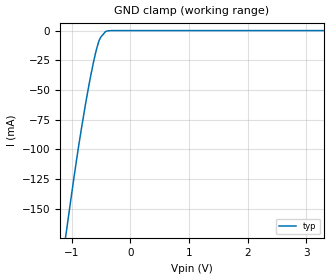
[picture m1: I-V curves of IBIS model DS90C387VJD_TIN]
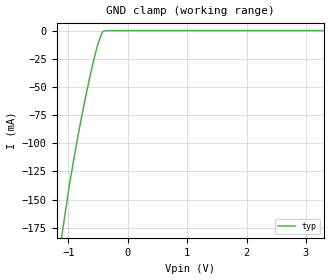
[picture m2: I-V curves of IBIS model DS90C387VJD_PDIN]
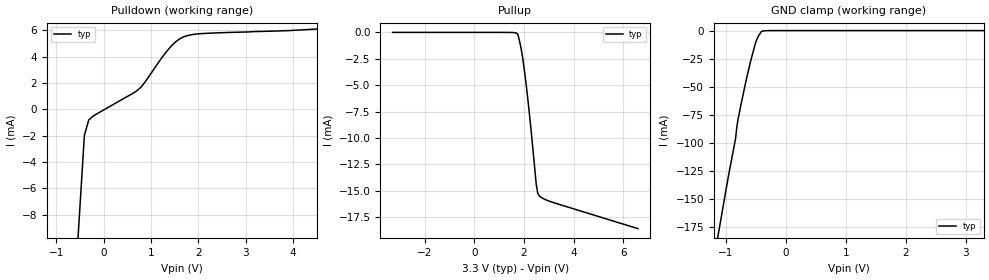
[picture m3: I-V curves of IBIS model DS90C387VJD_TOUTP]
|   National Semiconductor Corporation
|   Interface Products Group
|   IBIS Model of Channel Link Transmitter
|   100VJD TQFP
[IBIS Ver]   2.1
[Comment char]  |_char
[File name]   c387vjd.ibs
[File Rev]   2.0
[Date]   1/10/2000
[Source]   File originated at National Semiconductor Corporation.
   Interface Group/Analog Division. All data based on
   Empirical Measurements(Bench).
[Notes]   File created by CW.
   Revision 1: The original model
   Revision 2: Change "vdiff" values from "NA" to 0.1;
   Corrected "Ramp" rate data.
[Disclaimer]
(C) Copyright National Semiconductor Corporation 1999
   All rights reserved
   National Semiconductor Corporation hereby grants
the user of this IBIS model a non-exclusive, nontransferable
license to use this IBIS model under the following terms.
Before using this IBIS model, the user should read this
license.  If the user does not accept these terms,  the
IBIS model should be returned to National within 30 days.
   The user is granted this license only to use the
IBIS model and is not granted rights to sell, load, rent,
lease or license the IBIS model in whole or in part, or in
modified form to anyone other than user. User may modify
the IBIS model to suit its specific applications but rights
to derivative works and such modifications shall belong to
National.
   This IBIS model is provided on an "AS IS" basis and
National makes absolutely no warranty with respect to the
information contained herein. NATIONAL DISCLAIMS AND CUSTOMER
WAIVES ALL WARRANTIES, EXPRESS OR IMPLIED, INCLUDING
WARRANTIES OF MERCHANTABILITY OR FITNESS FOR A PARTICULAR
PURPOSE. The entire risk as to quality and performance is
with the Customer. ACCORDINGLY, IN NO EVENT SHALL THE
COMPANY BE LIABLE FOR ANY DAMAGES, WHETHER IN CONTRACT OR
TORT,INCLUDING ANY LOST PROFITS OR OTHER INCIDENTAL,
CONSEQUENTIAL, EXEMPLARY, OR PUNITIVE DAMAGES ARISING OUT
OF THE USE OR APPLICATION OF THE IBIS model provided in
this package. Further, National reserves the right to make
changes without notice to any product herein to improve
reliability, function, or design. National does not convey
any license under patent rights or any other intellectual
property rights, including those of third parties.
   National is not obligated to provide maintenance or support
for the licensed IBIS model.
Contact National at ATTN:INTERFACE APPLICATIONS/IBIS MODELS.
2900 Semiconductor Drive, M/S A2595, Santa Clara, CA 95052-8090
|!!!Please note pre-emphasis feature is NOT modeled!!!
[Copyright]   Copyright 1999, National Semiconductor, All Rights Reserved
[Component]   DS90C387VJD
[Manufacturer]  National Semiconductor Corp
[Package]
|   typ   min   max
R_pkg   64.20m   NA   NA
L_pkg   2.491nH   NA   NA
C_pkg   0.3380pF   NA   NA
[Pin]   signal_name   model_name   R_pin   L_pin   C_pin
1   TxING11   DS90C387VJD_TIN   70.72m  2.917n   0.3789p
2   TxING10   DS90C387VJD_TIN   70.51m  2.771n   0.3776p
3   TxINR17   DS90C387VJD_TIN   68.62m  2.713n   0.3658p
4   TxINR16   DS90C387VJD_TIN   67.20m  2.650n   0.3568p
5   TxINR15   DS90C387VJD_TIN   65.58m  2.545n   0.3467p
6   TxINR14   DS90C387VJD_TIN   64.85m  2.496n   0.3421p
7   TxINR13   DS90C387VJD_TIN   63.40m  2.419n   0.3328p
8   TxINR12   DS90C387VJD_TIN   62.50m  2.437n   0.3272p
9   TxINR11   DS90C387VJD_TIN   61.19m  2.376n   0.3192p
10   TxINR10   DS90C387VJD_TIN   60.16m  2.276n   0.3127p
11   TxCLKIN   DS90C387VJD_TIN   59.45m  2.239n   0.3083p
12   PLLVCC   POWER   58.73m  2.205n   0.3038p
13   GND   GND   59.19m  2.179n   0.3067p
14   PRE   DS90C387VJD_PDIN   58.73m  2.205n   0.3038p
15   PLLSEL   DS90C387VJD_PDIN   59.45m  2.239n   0.3083p
16   PLLGND   GND   60.16m  2.276n   0.3127p
17   PLLGND   GND   61.19m  2.376n   0.3192p
18   PLLVCC   POWER   62.50m  2.437n   0.3272p
19   PLLGND   GND   63.40m  2.419n   0.3328p
20   R_FB   DS90C387VJD_PDIN   64.85m  2.496n   0.3421p
21   R_FDE   DS90C387VJD_PDIN   65.58m  2.545n   0.3467p
22   PD*   DS90C387VJD_PDIN   67.20m  2.650n   0.3568p
23   DUAL   DS90C387VJD_PDIN   68.62m  2.713n   0.3658p
24   BAL   DS90C387VJD_PDIN   70.51m  2.771n   0.3776p
25   LVDSGND   GND   70.72m  2.917n   0.3789p
26   TxCLKOUT2+   DS90C387VJD_TOUTP   70.72m  2.917n   0.3789p
27   TxCLKOUT2-   DS90C387VJD_TOUTM   70.51m  2.771n   0.3776p
28   TxOUTA7+   DS90C387VJD_TOUTP   68.62m  2.713n   0.3658p
29   TxOUTA7-   DS90C387VJD_TOUTM   67.20m  2.650n   0.3568p
30   LVDSVCC   POWER   65.58m  2.545n   0.3467p
31   TxOUTA6+   DS90C387VJD_TOUTP   64.85m  2.496n   0.3421p
32   TxOUTA6-   DS90C387VJD_TOUTM   63.40m  2.419n   0.3328p
33   TxOUTA5+   DS90C387VJD_TOUTP   62.50m  2.437n   0.3272p
34   TxOUTA5-   DS90C387VJD_TOUTM   61.19m  2.376n   0.3192p
35   LVDSGND   GND   60.16m  2.276n   0.3127p
36   TxOUTA4+   DS90C387VJD_TOUTP   59.45m  2.239n   0.3083p
37   TxOUTA4-   DS90C387VJD_TOUTM   58.73m  2.205n   0.3038p
38   TxOUTA3+   DS90C387VJD_TOUTP   59.19m  2.179n   0.3067p
39   TxOUTA3-   DS90C387VJD_TOUTM   58.73m  2.205n   0.3038p
40   LVDSVCC   POWER   59.45m  2.239n   0.3083p
41   TxCLKOUT1+   DS90C387VJD_TOUTP   60.16m  2.276n   0.3127p
42   TxCLKOUT1-   DS90C387VJD_TOUTM   61.19m  2.376n   0.3192p
43   LVDSGND   GND   62.50m  2.437n   0.3272p
44   TxOUTA2+   DS90C387VJD_TOUTP   63.40m  2.419n   0.3328p
45   TxOUTA2-   DS90C387VJD_TOUTM   64.85m  2.496n   0.3421p
46   TxOUTA1+   DS90C387VJD_TOUTP   65.58m  2.545n   0.3467p
47   TxOUTA1-   DS90C387VJD_TOUTM   67.20m  2.650n   0.3568p
48   LVDSVCC   POWER   68.62m  2.713n   0.3658p
49   TxOUTA0+   DS90C387VJD_TOUTP   70.51m  2.771n   0.3776p
50   TxOUTA0-   DS90C387VJD_TOUTM   70.72m  2.917n   0.3789p
51   LVDSGND   GND   70.72m  2.917n   0.3789p
52   GND   GND   70.51m  2.771n   0.3776p
53   VCC   POWER   68.62m  2.713n   0.3658p
54   HSYNC   DS90C387VJD_TIN   67.20m  2.650n   0.3568p
55   VSYNC   DS90C387VJD_TIN   65.58m  2.545n   0.3467p
56   DE   DS90C387VJD_TIN   64.85m  2.496n   0.3421p
57   TxINB27   DS90C387VJD_TIN   63.40m  2.419n   0.3328p
58   TxINB26   DS90C387VJD_TIN   62.50m  2.437n   0.3272p
59   TxINB25   DS90C387VJD_TIN   61.19m  2.376n   0.3192p
60   TxINB24   DS90C387VJD_TIN   60.16m  2.276n   0.3127p
61   TxINB23   DS90C387VJD_TIN   59.45m  2.239n   0.3083p
62   TxINB22   DS90C387VJD_TIN   58.73m  2.205n   0.3038p
63   TxINB21   DS90C387VJD_TIN   59.19m  2.179n   0.3067p
64   TxINB20   DS90C387VJD_TIN   58.73m  2.205n   0.3038p
65   TxING27   DS90C387VJD_TIN   59.45m  2.239n   0.3083p
66   TxING26   DS90C387VJD_TIN   60.16m  2.276n   0.3127p
67   VCC   POWER   61.19m  2.376n   0.3192p
68   GND   GND   62.50m  2.437n   0.3272p
69   TxING25   DS90C387VJD_TIN   63.40m  2.419n   0.3328p
70   TxING24   DS90C387VJD_TIN   64.85m  2.496n   0.3421p
71   TxING23   DS90C387VJD_TIN   65.58m  2.545n   0.3467p
72   TxING22   DS90C387VJD_TIN   67.20m  2.650n   0.3568p
73   TxING21   DS90C387VJD_TIN   68.62m  2.713n   0.3658p
74   TxING20   DS90C387VJD_TIN   70.51m  2.771n   0.3776p
75   TxINR27   DS90C387VJD_TIN   70.72m  2.917n   0.3789p
76   TxINR26   DS90C387VJD_TIN   70.72m  2.917n   0.3789p
77   TxINR25   DS90C387VJD_TIN   70.51m  2.771n   0.3776p
78   TxINR24   DS90C387VJD_TIN   68.62m  2.713n   0.3658p
79   TxINR23   DS90C387VJD_TIN   67.20m  2.650n   0.3568p
80   TxINR22   DS90C387VJD_TIN   65.58m  2.545n   0.3467p
81   TxINR21   DS90C387VJD_TIN   64.85m  2.496n   0.3421p
82   VCC   POWER   63.40m  2.419n   0.3328p
83   GND   GND   62.50m  2.437n   0.3272p
84   TxINR20   DS90C387VJD_TIN   61.19m  2.376n   0.3192p
85   TxINB17   DS90C387VJD_TIN   60.16m  2.276n   0.3127p
86   TxINB16   DS90C387VJD_TIN   59.45m  2.239n   0.3083p
87   TxINB15   DS90C387VJD_TIN   58.73m  2.205n   0.3038p
88   TxINB14   DS90C387VJD_TIN   59.19m  2.179n   0.3067p
89   TxINB13   DS90C387VJD_TIN   58.73m  2.205n   0.3038p
90   TxINB12   DS90C387VJD_TIN   59.45m  2.239n   0.3083p
91   TxINB11   DS90C387VJD_TIN   60.16m  2.276n   0.3127p
92   TxINB10   DS90C387VJD_TIN   61.19m  2.376n   0.3192p
93   TxING17   DS90C387VJD_TIN   62.50m  2.437n   0.3272p
94   TxING16   DS90C387VJD_TIN   63.40m  2.419n   0.3328p
95   TxING15   DS90C387VJD_TIN   64.85m  2.496n   0.3421p
96   TxING14   DS90C387VJD_TIN   65.58m  2.545n   0.3467p
97   VCC   POWER   67.20m  2.650n   0.3568p
98   GND   GND   68.62m  2.713n   0.3658p
99   TxING13   DS90C387VJD_TIN   70.51m  2.771n   0.3776p
100   TxING12   DS90C387VJD_TIN   70.72m  2.917n   0.3789p
[Diff_pin]   inv_pin   vdiff   tdelay_typ   tdelay_min   tdelay_max
| The '+' pin is Diff_pin and the '-' pin is the inv_pin
26   27   0.1   0 0 0
28   29   0.1   0 0 0
31   32   0.1   0 0 0
33   34   0.1   0 0 0
36   37   0.1   0 0 0
38   39   0.1   0 0 0
41   42   0.1   0 0 0
44   45   0.1   0 0 0
46   47   0.1   0 0 0
49   50   0.1   0 0 0
| Models and submodels in the file (4): DS90C387VJD_TIN (Input), DS90C387VJD_PDIN (Input), DS90C387VJD_TOUTP (3-state), DS90C387VJD_TOUTM (3-state)
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|   Driver Input  MODEL
[Model]   DS90C387VJD_TIN
Model_type   Input
|Signals   TxINR10 ~ TxINR17, TxINR20 ~ TxINR27, TxING10 ~ TxING17,
|   TxING20 ~ TxING27, TxING10 ~ TxING17, TxING20 ~ TxING27,
|   TxCLKIN, HSYNC, VSYNC, DE, PRE, PLLSEL, R_FB, R_FDE, DUAL, BAL
Vinh = 2.0
Vinl = 0.8
|   typ   min   max
C_comp   5.217pF   NA   NA
|   typ   min   max
[Temperature Range]   25.0   NA   NA
[Voltage range]   3.3V   3.0V   3.6V
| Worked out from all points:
|   GND clamp passes 1 mA (typ) near -0.43 V on its own axis
[Power_clamp]
| Note that the[POWER_clamp]voltage table is referenced to Vcc
| and is calculated using Vtable=Vcc - Vmeasured.
|Voltage   I(typ)   I(min)   I(max)
-3V       0A         NA         NA
3V        0A         NA         NA
[GND_clamp]
|Voltage   I(typ)   I(min)   I(max)
-3.3V     -946.6mA   NA         NA
-1.001V   -136.5mA   NA         NA
-920.1mV  -108.8mA   NA         NA
-838.9mV  -83.09mA   NA         NA
-736.2mV  -53.35mA   NA         NA
-675.7mV  -37.16mA   NA         NA
-634.4mV  -27.34mA   NA         NA
-572.4mV  -14.46mA   NA         NA
-531.6mV  -7.937mA   NA         NA
-429.8mV  -1.026mA   NA         NA
-285.7mV  -7.334uA   NA         NA
3.3V      -100.8nA   NA         NA
|   Driver PWRDWN* Input  MODEL
[Model]   DS90C387VJD_PDIN
Model_type   Input
|Signals   PD*
Vinh = 2.0
Vinl = 0.8
|   typ   min   max
C_comp   5.277pF   NA   NA
|   typ   min   max
[Temperature Range]   25.0   NA   NA
[Voltage range]   3.3V   3.0V   3.6V
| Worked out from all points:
|   GND clamp passes 1 mA (typ) near -0.42 V on its own axis
[Power_clamp]
| Note that the[POWER_clamp]voltage table is referenced to Vcc
| and is calculated using Vtable=Vcc - Vmeasured.
|Voltage   I(typ)   I(min)   I(max)
-3V       0A         NA         NA
3V        0A         NA         NA
[GND_clamp]
|Voltage   I(typ)   I(min)   I(max)
-3.3V     -959.1mA   NA         NA
-1V       -143mA     NA         NA
-982mV    -136.5mA   NA         NA
-920.1mV  -117.4mA   NA         NA
-818.3mV  -87.77mA   NA         NA
-715.5mV  -60.23mA   NA         NA
-613.7mV  -35.12mA   NA         NA
-552.2mV  -21.69mA   NA         NA
-490.3mV  -9.998mA   NA         NA
-428.8mV  -1.679mA   NA         NA
-408.2mV  -422.1uA   NA         NA
3.3V      0A         NA         NA
|   Driver Output(+)  MODEL
[Model]   DS90C387VJD_TOUTP
Model_type   3-state
| Signals   TxOUTA0+ ~ TxOUTA7+; TxCLKOUT1+; TxCLKOUT2+
Vmeas = 1.2V   |This is 0.0v differential on ouput
Cref = 5pF   |Timing specification test load capacitance value
Rref = 50
Vref = 1.2
| variable   typ   min   max
C_comp   5.074pF   NA   NA
|   typ   min   max
[Temperature Range]   25.0   NA   NA
[Voltage range]   3.3V   3.0V   3.6V
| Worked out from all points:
|   slope of the pulldown table from 0 to 0.495 V, typ, clamps not added: 489 ohm
|   GND clamp passes 1 mA (typ) near -0.41 V on its own axis
[Pulldown]
| Voltage   I(typ)   I(min)   I(max)
-3.3V     -169.3mA   NA         NA
-499.6mV  -7.251mA   NA         NA
-408.6mV  -1.987mA   NA         NA
-317.2mV  -816.7uA   NA         NA
-225.7mV  -523.9uA   NA         NA
786.3mV   1.673mA    NA         NA
1.428V    4.807mA    NA         NA
1.704V    5.521mA    NA         NA
1.98V     5.716mA    NA         NA
2.439V    5.802mA    NA         NA
4.5V      6.085mA    NA         NA
6.6V      6.199mA    NA         NA
[Pullup]
| Note that the[Pullup]voltage table is referenced to Vcc
| and is calculated using Vtable=Vcc - Vmeasured.
|Voltage   I(typ)   I(min)   I(max)
-3.3V     0A         NA         NA
1.684V    -48.2uA    NA         NA
1.751V    -184.9uA   NA         NA
1.819V    -808.9uA   NA         NA
1.886V    -1.554mA   NA         NA
2.02V     -3.66mA    NA         NA
2.223V    -7.817mA   NA         NA
2.493V    -14.39mA   NA         NA
2.558V    -15.28mA   NA         NA
2.694V    -15.63mA   NA         NA
3.098V    -16.06mA   NA         NA
6.6V      -18.59mA   NA         NA
[GND_clamp]
| Outputs in Tri-state.
| Voltage   I(typ)   I(min)   I(max)
-3.3V     -852.7mA   NA         NA
-1.001V   -143.3mA   NA         NA
-838.4mV  -96.78mA   NA         NA
-816.8mV  -86.45mA   NA         NA
-797.1mV  -79.34mA   NA         NA
-654.5mV  -42.85mA   NA         NA
-593.5mV  -28.73mA   NA         NA
-511.4mV  -12.19mA   NA         NA
-450.9mV  -4.248mA   NA         NA
-408.6mV  -945.1uA   NA         NA
-265.5mV  -6.81uA    NA         NA
3.3V      0A         NA         NA
[POWER_clamp]
| Note that the[POWER_clamp]voltage table is referenced to Vcc
| and is calculated using Vtable=Vcc - Vmeasured.
| Outputs in Tri-state.
|Voltage   I(typ)   I(min)   I(max)
-3V       0A         NA         NA
3V        0A         NA         NA
[Ramp]
| Note: Ramp rate measured on single-ended Driver Output.
|   typ   min   max
dV/dt_r   180.0m/0.510n   NA   NA
dV/dt_f   115.0m/0.163n   NA   NA
R_load = 100Ohm | Note: This 100 Ohm is across the two driver output
